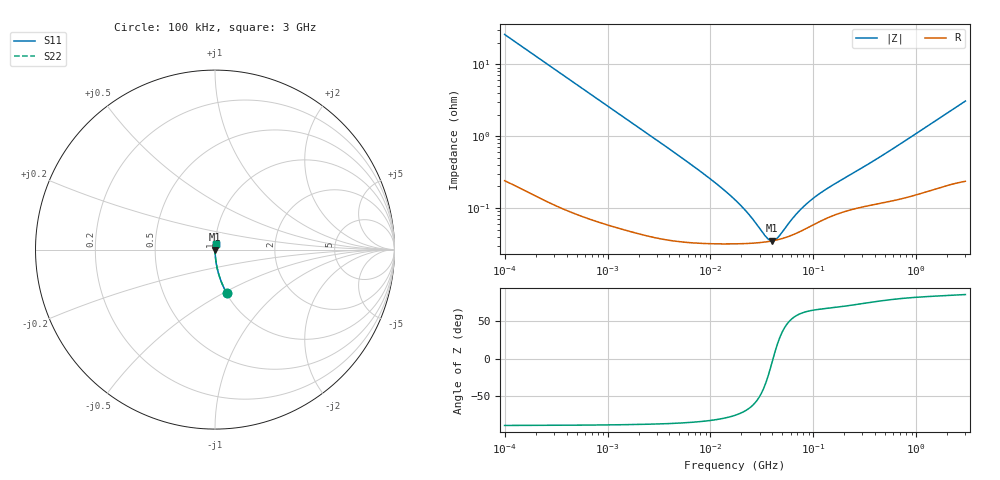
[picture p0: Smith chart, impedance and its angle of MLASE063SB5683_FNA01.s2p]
! MLASE063SB5683_FNA01  S-PARAMETER MODEL  ( Standard Model )
! Model Generated by TAIYO YUDEN Corporation (http://www.ty-top.com)
! Version 1.0
! TAIYO YUDEN Control No. 220601
! Copyright(c) 2013 TAIYO YUDEN CO.,LTD. All Rights Reserved.
! Product Description (link to TY-COMPAS)
! https://ds.yuden.co.jp/TYCOMPAS/or/detail?pn=MLASE063SB5683KFNA01&u=M
! Products Name : Multilayer Ceramic Capacitors
! Characteristics :
!  Capacitance : 0.068 [uF] , Rated Voltage : 16 [V] , TCC : X5R
!  Case Size : 0.6 x 0.3 / 0.024 x 0.012 [mm/inch] , Thickness : 0.3 / 0.012 [mm/inch]
!  (Conditions: Temperature = 25 [degC] , DC Bias Voltage = 0 [V])
! External Node Assignments :
!  1  o---| |---o  2
! GND o---------o GND
! Frequency Range : 100kHz  -  3GHz  [ 401 STEP ]
# MHZ S RI R 50
! Freq[MHz].  S11 Real  S11 Imag  S21 Real  S21 Imag  S12 Real  S12 Imag  S22 Real  S22 Imag
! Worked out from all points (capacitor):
!   401 points, 100 kHz to 3 GHz, reference 50 ohm
!   read as one part in series: C = 61 nF near 105.3 kHz
!   lowest |Z| = 35 mohm at 39.51 MHz (marker M1)
!   series resonance near 40.61 MHz, so ESL is about 250 pH
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0.1  0.0655 -0.2429  0.9345 0.2429  0.9345 0.2429  0.0655 -0.2429
0.151038  0.0307 -0.1673  0.9693 0.1673  0.9693 0.1673  0.0307 -0.1673
0.222319  0.015 -0.1158  0.985 0.1158  0.985 0.1158  0.015 -0.1158
0.344552  0.00677 -0.0756  0.9932 0.0756  0.9932 0.0756  0.00677 -0.0756
0.562235  0.00295 -0.0466  0.9971 0.0466  0.9971 0.0466  0.00295 -0.0466
1.18716  0.00104 -0.0222  0.999 0.0222  0.999 0.0222  0.00104 -0.0222
3.161081  0.000447 -0.00838  0.9996 0.00838  0.9996 0.00838  0.000447 -0.00838
9.574722  0.000326 -0.00264  0.9997 0.00264  0.9997 0.00264  0.000326 -0.00264
13.38544  0.00032 -0.00178  0.9997 0.00178  0.9997 0.00178  0.00032 -0.00178
17.7727  0.000319 -0.00122  0.9997 0.00122  0.9997 0.00122  0.000319 -0.00122
24.21403  0.000323 -0.000713  0.9997 0.000713  0.9997 0.000713  0.000323 -0.000713
34.73492  0.000338 -0.000207  0.9997 0.000207  0.9997 0.000207  0.000338 -0.000207
37.52708  0.000344 -0.000104  0.9997 0.000104  0.9997 0.000104  0.000344 -0.000104
39.51212  0.000348 -3.61e-05  0.9997 3.61e-05  0.9997 3.61e-05  0.000348 -3.61e-05
41.60216  0.000353 3.16e-05  0.9996 -3.16e-05  0.9996 -3.16e-05  0.000353 3.16e-05
44.94634  0.000362 0.000133  0.9996 -0.000133  0.9996 -0.000133  0.000362 0.000133
67.88584  0.000444 0.000686  0.9996 -0.000686  0.9996 -0.000686  0.000444 0.000686
81.30716  0.000503 0.000939  0.9995 -0.000939  0.9995 -0.000939  0.000503 0.000939
97.38194  0.000575 0.0012  0.9994 -0.0012  0.9994 -0.0012  0.000575 0.0012
143.341  0.000751 0.00181  0.9992 -0.00181  0.9992 -0.00181  0.000751 0.00181
547.5153  0.00127 0.00609  0.9987 -0.00609  0.9987 -0.00609  0.00127 0.00609
3000  0.00329 0.0306  0.9967 -0.0306  0.9967 -0.0306  0.00329 0.0306
